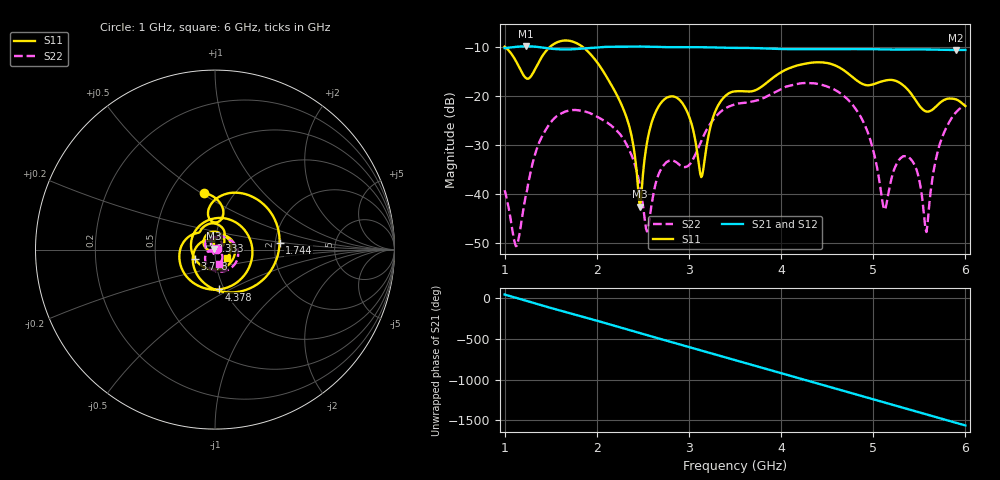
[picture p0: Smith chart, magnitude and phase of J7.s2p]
!Agilent Technologies,E8364B,MY43040528,A.07.50.67
!Agilent E8364B: A.07.50.67
!Date: Sunday, March 01, 2026 15:27:19
!Correction: S11(Full 2 Port(1,2))
!S21(Full 2 Port(1,2))
!S12(Full 2 Port(1,2))
!S22(Full 2 Port(1,2))
!S2P File: Measurements: S11, S21, S12, S22:
# Hz S  dB  R 50
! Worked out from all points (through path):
!   451 points, 1 GHz to 6 GHz, reference 50 ohm
!   highest |S21| = -9.74 dB at 1.233 GHz (marker M1); lowest = -10.5 dB at 5.9 GHz (marker M2)
!   group delay of S21, straight-line fit = 892 ps
!   lowest |S11| = -42.6 dB at 2.467 GHz (marker M3), VSWR 1.01, Z = 49.5 + j0.528 ohm
!   |S11| at or under -10 dB: 1.011 GHz to 1.485 GHz (474.5 MHz wide, 38 % of centre); 1.856 GHz to end of sweep
!   |S22| runs from -50.7 to -17.3 dB; largest |S21 - S12| = 0.0014
!   S11 on the Smith chart (normalised r, x): 1 GHz: 0.73, +0.51; 1.744 GHz: 2.11, +0.18; 2.333 GHz: 0.94, +0.10; 3.778 GHz: 0.79, -0.08; 4.378 GHz: 0.94, -0.44; 6 GHz: 1.14, -0.10
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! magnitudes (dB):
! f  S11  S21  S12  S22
! 1 GHz  -9.8  -10.1  -10.2  -39.2
! 1.122 GHz  -12.8  -9.9  -9.9  -50.7
! 1.233 GHz  -16.3  -9.7  -9.8  -40.0
! 1.744 GHz  -8.8  -10.4  -10.4  -22.8
! 1.844 GHz  -9.8  -10.2  -10.2  -23.0
! 2.333 GHz  -24.9  -9.8  -9.8  -30.2
! 2.467 GHz  -42.6  -9.8  -9.8  -38.2
! 2.544 GHz  -29.6  -9.8  -9.9  -47.7
! 2.667 GHz  -22.2  -9.9  -9.9  -36.2
! 2.933 GHz  -21.5  -9.9  -10.0  -34.4
! 3.133 GHz  -36.5  -9.9  -10.0  -29.2
! 3.5 GHz  -19.0  -10.1  -10.1  -21.6
! 3.778 GHz  -18.2  -10.2  -10.2  -20.6
! 4.344 GHz  -13.1  -10.3  -10.4  -17.3
! 4.378 GHz  -13.0  -10.3  -10.4  -17.4
! 4.833 GHz  -16.9  -10.3  -10.4  -23.2
! 5.167 GHz  -16.6  -10.4  -10.4  -39.7
! 5.389 GHz  -18.9  -10.4  -10.4  -32.5
! 5.578 GHz  -23.1  -10.4  -10.4  -47.8
! 5.7 GHz  -21.7  -10.5  -10.5  -31.3
! 5.9 GHz  -20.6  -10.5  -10.5  -23.2
! 6 GHz  -22.0  -10.5  -10.5  -21.6
